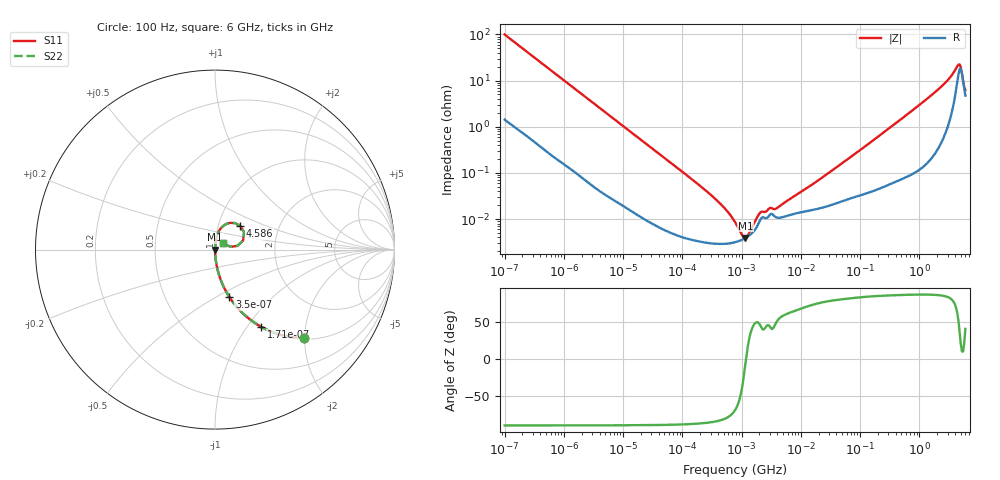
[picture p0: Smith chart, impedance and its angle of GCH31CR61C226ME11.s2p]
!Murata Part Number: GCH31CR61C226ME11
!These Parameters are Measured in Series Mode Connection
!Data Generated on Jun 19, 2026
!  o--ll--o
!Port1  Port2
!  o------o
!Operation Temp=25[degC], DC Bias Voltage=0[V]
!Freq. Start=100[Hz] Stop=6[GHz] 401[Steps]
# Hz S RI R 50
!Freq.(Hz) S11(Real) S11(Imag) S21(Real) S21(Imag) S12(Real) S12(Imag) S22(Real) S22(Imag)
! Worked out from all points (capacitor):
!   401 points, 100 Hz to 6 GHz, reference 50 ohm
!   read as one part in series: C = 15.9 uF near 109 Hz
!   lowest |Z| = 3.9 mohm at 1.159 MHz (marker M1)
!   series resonance near 1.187 MHz, so ESL is about 1.1 nH
!   S11 on the Smith chart (normalised r, x): 100 Hz: 1.03, -1.99; 171 Hz: 1.02, -1.17; 350 Hz: 1.01, -0.58; 4.586 GHz: 1.27, +0.35; 6 GHz: 1.09, +0.08
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100  0.4986 -0.4929  0.5014 0.4929  0.5014 0.4929  0.4986 -0.4929
171  0.2583 -0.4305  0.7417 0.4305  0.7417 0.4305  0.2583 -0.4305
350  0.0799 -0.2639  0.9201 0.2639  0.9201 0.2639  0.0799 -0.2639
784  0.0183 -0.1269  0.9817 0.1269  0.9817 0.1269  0.0183 -0.1269
2008  0.00339 -0.0508  0.9966 0.0508  0.9966 0.0508  0.00339 -0.0508
40335  7.31e-05 -0.00262  0.9999 0.00262  0.9999 0.00262  7.31e-05 -0.00262
276587  3.04e-05 -0.000368  1 0.000368  1 0.000368  3.04e-05 -0.000368
774597  3.15e-05 -8.04e-05  1 8.04e-05  1 8.04e-05  3.15e-05 -8.04e-05
1159002  3.88e-05 -4.3e-06  1 4.3e-06  1 4.3e-06  3.88e-05 -4.3e-06
1658239  5.73e-05 6.42e-05  0.9999 -6.42e-05  0.9999 -6.42e-05  5.73e-05 6.42e-05
2169299  0.000106 9.86e-05  0.9999 -9.86e-05  0.9999 -9.86e-05  0.000106 9.86e-05
3103719  0.000129 0.000119  0.9999 -0.000119  0.9999 -0.000119  0.000129 0.000119
3882480  0.000108 0.000131  0.9999 -0.000131  0.9999 -0.000131  0.000108 0.000131
1.555665e7  0.000157 0.000537  0.9998 -0.000537  0.9998 -0.000537  0.000157 0.000537
3.124326e8  0.000647 0.00932  0.9994 -0.00932  0.9994 -0.00932  0.000647 0.00932
1.309207e9  0.00306 0.0388  0.9969 -0.0388  0.9969 -0.0388  0.00306 0.0388
2.802721e9  0.0157 0.0898  0.9843 -0.0898  0.9843 -0.0898  0.0157 0.0898
3.666503e9  0.0417 0.1283  0.9583 -0.1283  0.9583 -0.1283  0.0417 0.1283
4.193612e9  0.0851 0.149  0.9149 -0.149  0.9149 -0.149  0.0851 0.149
4.586474e9  0.141 0.1322  0.859 -0.1322  0.859 -0.1322  0.141 0.1322
5.016141e9  0.1562 0.0504  0.8438 -0.0504  0.8438 -0.0504  0.1562 0.0504
6e9  0.0465 0.0378  0.9535 -0.0378  0.9535 -0.0378  0.0465 0.0378
